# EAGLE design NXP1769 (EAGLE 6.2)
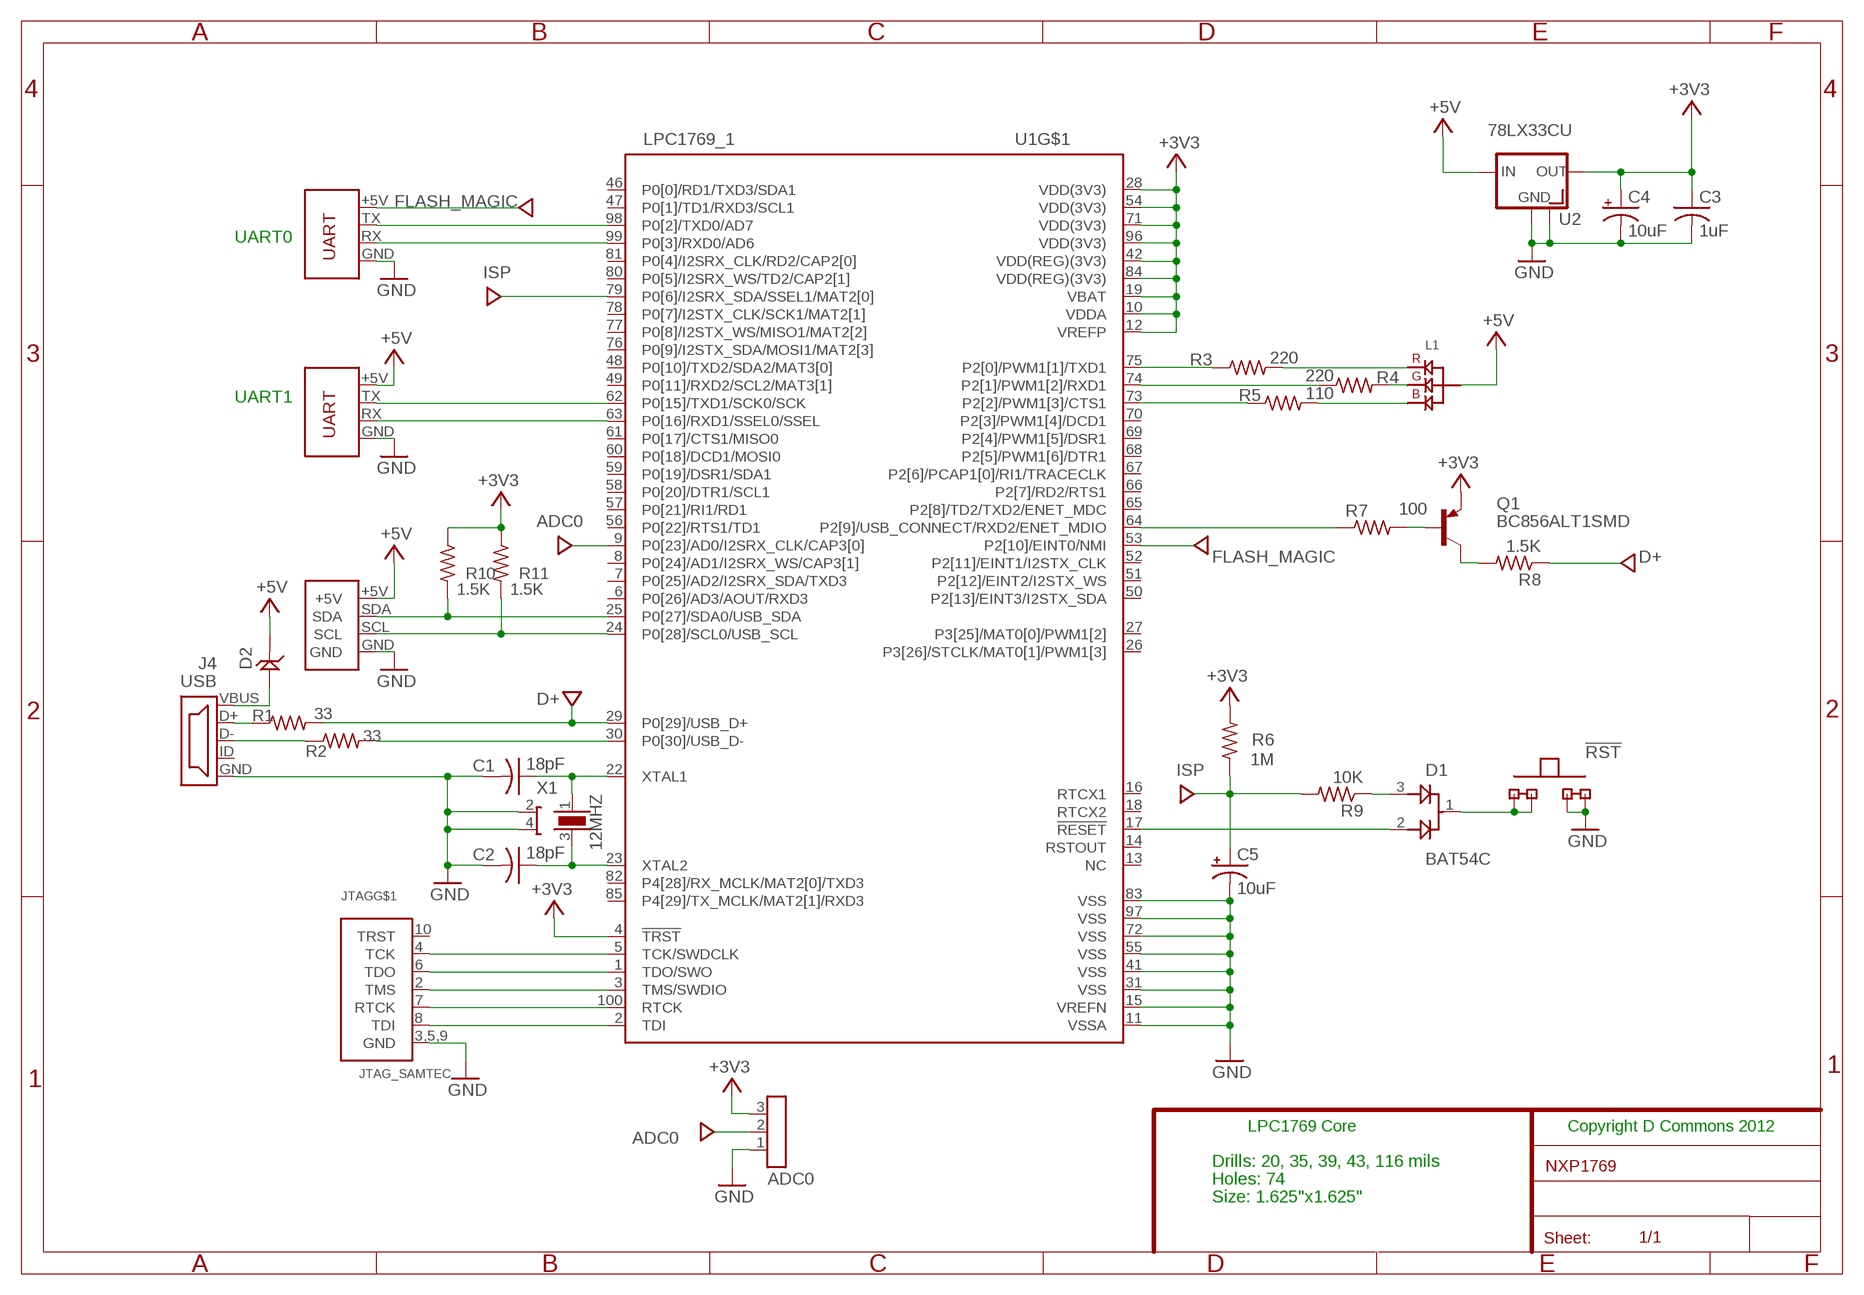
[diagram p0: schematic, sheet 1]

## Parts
!RST  SIDE_SWITCH  [COLLISION]
ADC0  1X3  [1X03]
C1  18pF  C-USC0805  [C0805]
C2  18pF  C-USC0805  [C0805]
C3  1uF  C-USC0805  [C0805]
C4  10uF  C_POL1206  [C1206P]
C5  10uF  C_POL1206  [C1206P]
D1  BAT54C  [SOT23-BAT54C]
D2  PMEG2005  [SOT23]
J1  ISNAP  [ISNAP]
J4  USB  [USB-MB-S]
JTAG  JTAG_SAMTEC  [2X10X0.5MM]
L1  RGB_ANODE  [3.2X2.7]
Q1  BC856ALT1SMD  [SOT23-BEC]
R1  33  R-US_R0805  [R0805]
R2  33  R-US_R0805  [R0805]
R3  220  R-US_R0805  [R0805]
R4  220  R-US_R0805  [R0805]
R5  110  R-US_R0805  [R0805]
R6  1M  R-US_R0805  [R0805]
R7  100  R-US_R0805  [R0805]
R8  1.5K  R-US_R0805  [R0805]
R9  10K  R-US_R0805  [R0805]
R10  1.5K  R-US_R0805  [R0805]
R11  1.5K  R-US_R0805  [R0805]
U1  LPC1769_1  [LQFP100-14X14]
U2  78LX33CU  [SOT89]
UART0  IMU_UART  [IMU_UART]
UART1  IMU_UART  [IMU_UART]
X1  12MHZ  16MHZ  [3.2X2.5_XTAL]

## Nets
!RESET: D1.2 U1.17(!RESET)
!RST_SW: !RST.A !RST.A@1(A) D1.1
+3V3 [+3V3]: ADC0.3 C3.1 C4.+ Q1.E R6.2 R10.1 R11.1 U1.4(!TRST) U1.10(VDDA) U1.12(VREFP) U1.19(VBAT) U1.28(VDD(3V3)) U1.42(VDD(REG)(3V3)) U1.54(VDD(3V3)) U1.71(VDD(3V3)) U1.84(VDD(REG)(3V3)) U1.96(VDD(3V3)) U2.1(OUT)
+5V [+5V]: D2.3(CATHODE) J1.+5V L1.A U2.3(IN) UART1.+5V
ADC0: ADC0.2 U1.9(P0[23]/AD0/I2SRX_CLK/CAP3[0])
BLUE: L1.B R5.2
D+: R1.2 R8.1 U1.29(P0[29]/USB_D+)
D-: R2.2 U1.30(P0[30]/USB_D-)
DD+: J4.D+ R1.1
DD-: J4.D- R2.1
FLASH_MAGIC: U1.53(P2[10]/EINT0/NMI) UART0.+5V
GND: !RST.B !RST.B@1(B) ADC0.1 C1.2 C2.2 C3.2 C4.- C5.- J1.GND J4.GND JTAG.3,5,9(GND) U1.11(VSSA) U1.15(VREFN) U1.31(VSS) U1.41(VSS) U1.55(VSS) U1.72(VSS) U1.83(VSS) U1.97(VSS) U2.2(GND) U2.4(GND1) UART0.GND UART1.GND X1.2(GND) X1.4(GND)
GREEN: L1.G R4.2
ISP: C5.+ R6.1 R9.2 U1.79(P0[6]/I2SRX_SDA/SSEL1/MAT2[0])
N$24: Q1.B R7.2
N$25: Q1.C R8.2
N$28: D1.3 R9.1
P2.0: R3.1 U1.75(P2[0]/PWM1[1]/TXD1)
P2.1: R4.1 U1.74(P2[1]/PWM1[2]/RXD1)
P2.2: R5.1 U1.73(P2[2]/PWM1[3]/CTS1)
RED: L1.R R3.2
RTCK: JTAG.7(RTCK) U1.100(RTCK)
RXD0: U1.99(P0[3]/RXD0/AD6) UART0.RX
RXD1: U1.63(P0[16]/RXD1/SSEL0/SSEL) UART1.RX
SCL: J1.SCL R11.2 U1.24(P0[28]/SCL0/USB_SCL)
SDA: J1.SDA R10.2 U1.25(P0[27]/SDA0/USB_SDA)
TCK: JTAG.4(TCK) U1.5(TCK/SWDCLK)
TDI: JTAG.8(TDI) U1.2(TDI)
TDO: JTAG.6(TDO) U1.1(TDO/SWO)
TMS: JTAG.2(TMS) U1.3(TMS/SWDIO)
TXD0: U1.98(P0[2]/TXD0/AD7) UART0.TX
TXD1: U1.62(P0[15]/TXD1/SCK0/SCK) UART1.TX
USB_EN: R7.1 U1.64(P2[9]/USB_CONNECT/RXD2/ENET_MDIO)
VBUS: D2.1(ANODE) J4.VBUS
XTAL1: C1.1 U1.22(XTAL1) X1.1(X0)
XTAL2: C2.1 U1.23(XTAL2) X1.3(X1)
Unconnected: J4.ID(UID) JTAG.10(TRST) U1.6(P0[26]/AD3/AOUT/RXD3) U1.7(P0[25]/AD2/I2SRX_SDA/TXD3) U1.8(P0[24]/AD1/I2SRX_WS/CAP3[1]) U1.13(NC) U1.14(RSTOUT) U1.16(RTCX1) U1.18(RTCX2) U1.20(P1[31]/SCK1/AD05) U1.21(P1[30]/AD4) U1.26(P3[26]/STCLK/MAT0[1]/PWM1[3]) U1.27(P3[25]/MAT0[0]/PWM1[2]) U1.32(P1[18]/PWM1[1]/CAP1[0]) U1.33(P1[19]/MCOA0/USB_PPWR/CAP1[1]) U1.34(P1[20]/MCI0/PWM1[2]/SCK0) U1.35(P1[21]/MCABORT/PWM1[3]/SSEL0) U1.36(P1[22]/MCOB0/MAT1[0]) U1.37(P1[23]/MCI1/PWM1[4]/MISO0) U1.38(P1[24]/MCI2/PWM1[5]/MOSI0) U1.39(P1[25]/MCOA1/MAT1[1]) U1.40(P1[26]/MCOB1/PWM1[6]/CAP0[0]) U1.43(P1[27]/CLKOUT/CAP0[1]) U1.44(P1[28]/MCOA2/PCAP1[0]/MAT0[0]) U1.45(P1[29]/MCOB2/PCAP1[1]/MAT0[1]) U1.46(P0[0]/RD1/TXD3/SDA1) U1.47(P0[1]/TD1/RXD3/SCL1) U1.48(P0[10]/TXD2/SDA2/MAT3[0]) U1.49(P0[11]/RXD2/SCL2/MAT3[1]) U1.50(P2[13]/EINT3/I2STX_SDA) U1.51(P2[12]/EINT2/I2STX_WS) U1.52(P2[11]/EINT1/I2STX_CLK) U1.56(P0[22]/RTS1/TD1) U1.57(P0[21]/RI1/RD1) U1.58(P0[20]/DTR1/SCL1) U1.59(P0[19]/DSR1/SDA1) U1.60(P0[18]/DCD1/MOSI0) U1.61(P0[17]/CTS1/MISO0) U1.65(P2[8]/TD2/TXD2/ENET_MDC) U1.66(P2[7]/RD2/RTS1) U1.67(P2[6]/PCAP1[0]/RI1/TRACECLK) U1.68(P2[5]/PWM1[6]/DTR1) U1.69(P2[4]/PWM1[5]/DSR1) U1.70(P2[3]/PWM1[4]/DCD1) U1.76(P0[9]/I2STX_SDA/MOSI1/MAT2[3]) U1.77(P0[8]/I2STX_WS/MISO1/MAT2[2]) U1.78(P0[7]/I2STX_CLK/SCK1/MAT2[1]) U1.80(P0[5]/I2SRX_WS/TD2/CAP2[1]) U1.81(P0[4]/I2SRX_CLK/RD2/CAP2[0]) U1.82(P4[28]/RX_MCLK/MAT2[0]/TXD3) U1.85(P4[29]/TX_MCLK/MAT2[1]/RXD3) U1.86(P1[17]/ENET_MDIO) U1.87(P1[16]/ENET_MDC) U1.88(P1[15]/ENET_REF_CLK) U1.89(P1[14]/ENET_RX_ER) U1.90(P1[10]/ENET_RXD1) U1.91(P1[9]/ENET_RXD0) U1.92(P1[8]/ENET_CRS) U1.93(P1[4]/ENET_TX_EN) U1.94(P1[1]/ENET_TXD1) U1.95(P1[0]/ENET_TXD0)

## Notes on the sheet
- UART0
- UART1
- LPC1769 Core | Copyright D Commons 2012
- Drills: 20, 35, 39, 43, 116 mils
- Holes: 74
- Size: 1.625"x1.625"

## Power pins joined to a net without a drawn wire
GND: J4.GND@1(GND) J4.GND@2(GND) J4.GND@3(GND) J4.GND@4(GND) JTAG.3,5,9@1(GND) JTAG.3,5,9@2(GND)

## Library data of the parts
!RST = 1_Motor:SIDE_SWITCH
ADC0 = 1_Dougs_custom:1X3
C1-C3 = 1_Dougs_custom:C-US: CAPACITOR, American symbol
C4 C5 = 1_Dougs_custom:C_POL1206
D1 = 1_Dougs_custom:BAT54C
D2 = 1_Dougs_custom:PMEG2005
J1 = 1_Dougs_custom:ISNAP
J4 = 1_Dougs_custom:USB: USB Connectors
JTAG = 1_Dougs_custom:JTAG_SAMTEC
L1 = 1_Dougs_custom:RGB_ANODE
Q1 = transistor-pnp:BC856*: PNP Transistror
R1-R11 = 1_Dougs_custom:R-US_: RESISTOR, American symbol
U1 = 1_linux:LPC1769_1: LPC1768 100 MHz 32-bit ARM Cortex-M3 based microcontroller featuring a high level of integration and low power consumption. 512 kB Flash, 64 kB SRAM, USB Device/Host/OTG, 2 CAN, DAC, Ethernet MarcVl - Datasheet available on www.nxp.com
U2 = 1_Dougs_custom:78LX33CU: VOLTAGE REGULATOR
UART0 UART1 = 1_Dougs_custom:IMU_UART
X1 = RF_lib:16MHZ

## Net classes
1 +5V: width 0.381 mm
2 +3V3: width 0.229 mm

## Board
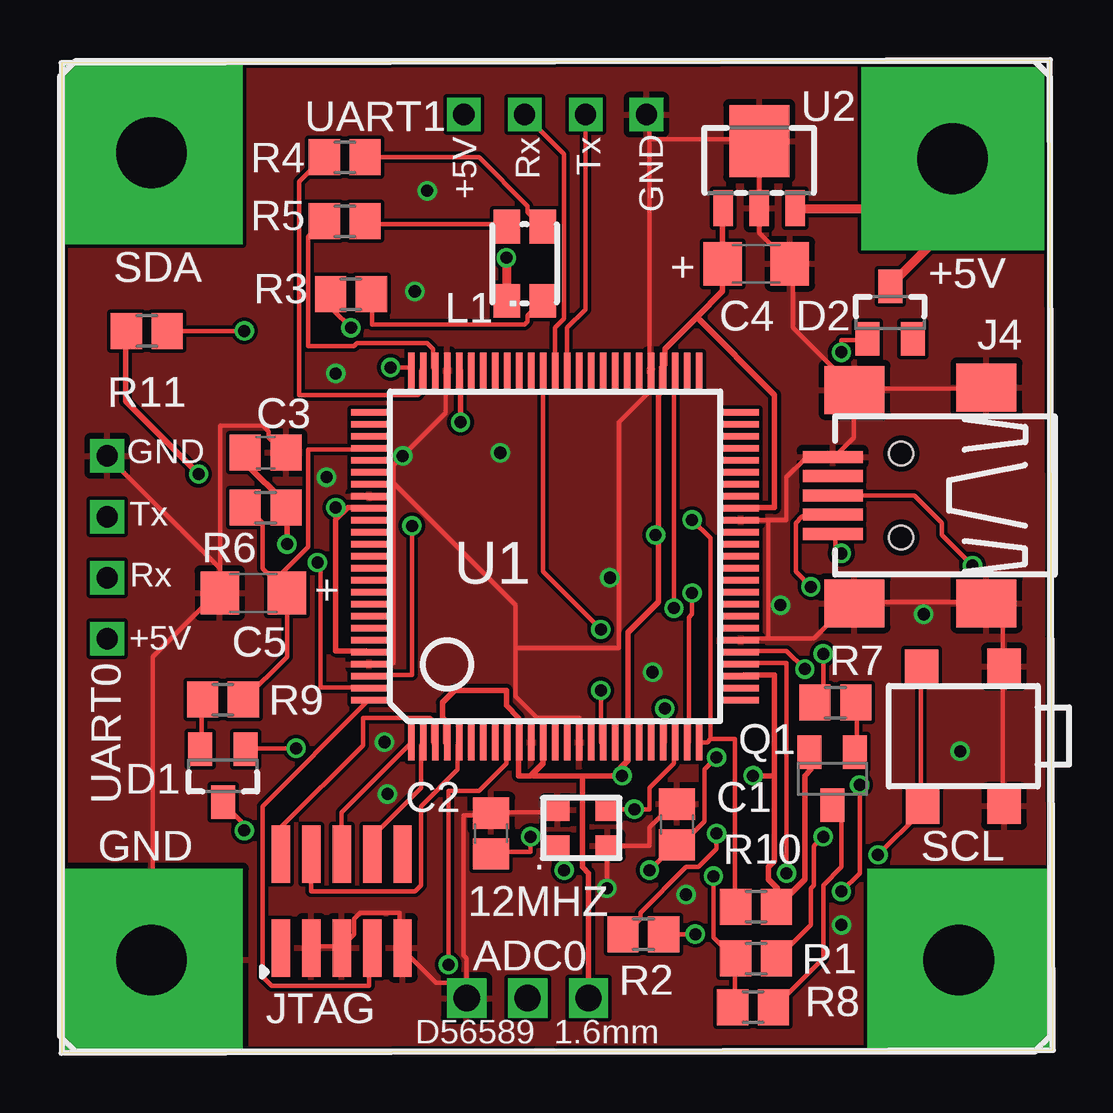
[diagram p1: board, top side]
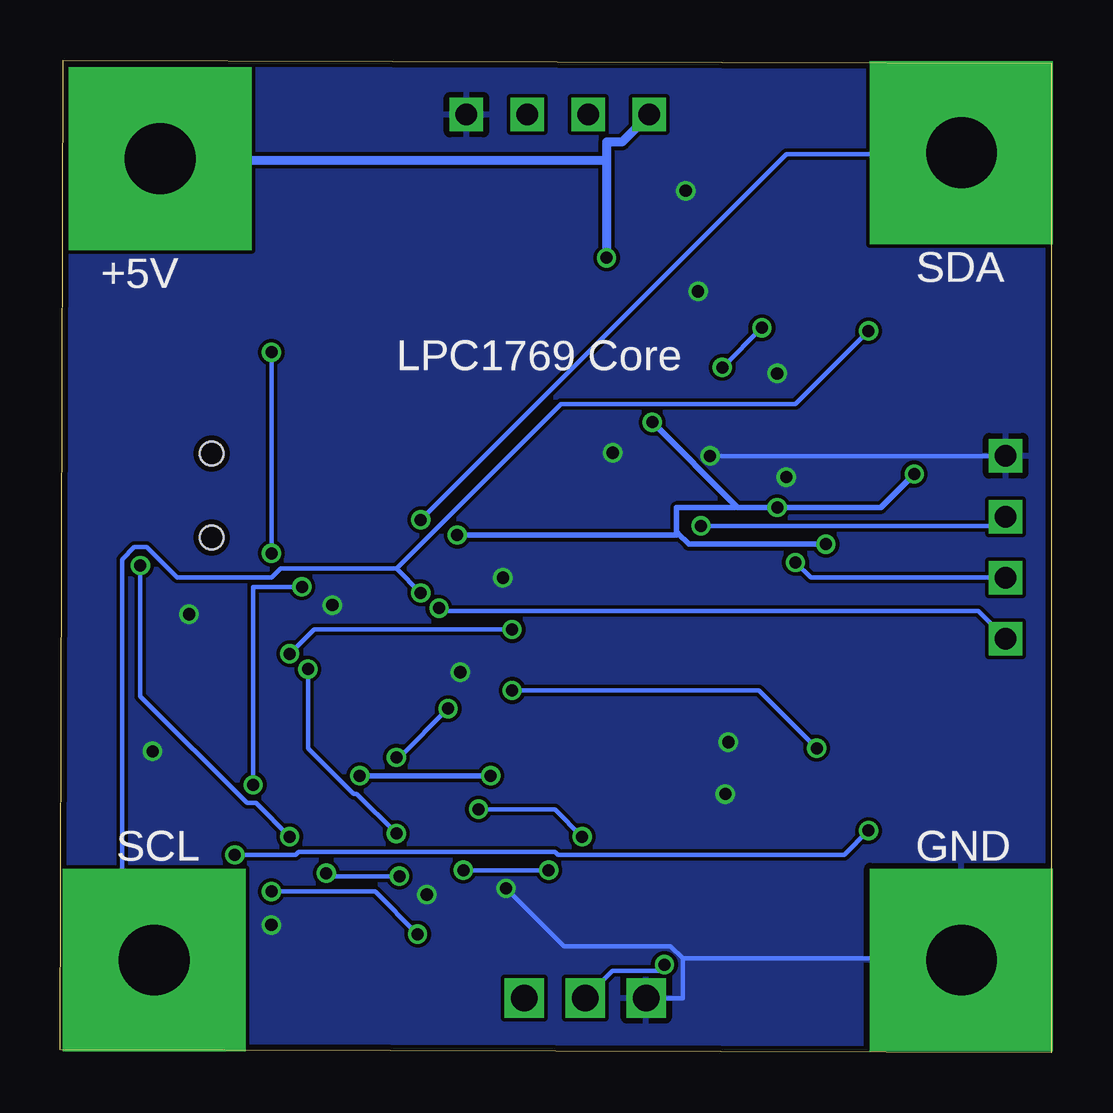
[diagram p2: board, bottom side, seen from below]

Size 41.33 x 41.39 mm. Coordinates in mm from the lower left corner, seen from the top.
Outline: 0,0 41.33,0.13 41.2,41.39 0,41.27 0,0
Copper layers (1*16): Top 0.035mm / dielectric 1.5mm / Bottom 0.035mm
Design rules: minimum track width 6mil, minimum drill 12mil, track to track 6mil, track to pad 6mil, pad to pad 6mil, via to via 6mil, smd to smd 0mil, copper to edge 10mil, drill to drill 10mil, minimum pad ring 10mil, minimum via ring 6mil, stop-mask expansion 2mil, vias tented up to drill 100mil, thermal gap 10mil

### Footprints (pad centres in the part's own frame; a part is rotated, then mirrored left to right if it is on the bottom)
COLLISION = smd 1.5 x 1.4: A 2.87,1.74; A@1 -2.9,1.7; B 2.9,-1.7; B@1 -2.91,-1.7
1X03 = drill 1.092 square: 1 -2.54,0; 2 0,0; 3 2.54,0
C0805 = smd 1.3 x 1.5: 1 -0.85,0; 2 0.85,0
C1206P = smd 1.6 x 1.8: + 1.4,0; - -1.4,0
SOT23-BAT54C = smd 1 x 1.4: 1 0,1.1; 2 -0.95,-1.1; 3 0.95,-1.1
SOT23 = smd 1 x 1.4: 1 -0.95,-1.1; 2 0.95,-1.1; 3 0,1.1
ISNAP = drill 2.946 pad 7.62 square: +5V 16.573,16.573; GND -16.828,-16.828; SCL 16.828,-16.828; SDA -16.828,16.828
USB-MB-S = smd 0.5 x 2.5: D+ 0,-9.25; D- 0.8,-9.25; GND -1.6,-9.25; ID -0.8,-9.25; VBUS 1.6,-9.25 | smd 2 x 2.5: GND@1 4.5,-2.842; GND@2 4.5,-8.342; GND@3 -4.5,-2.842; GND@4 -4.4,-8.342 | hole 0.991: -1.75,-6.4; 1.75,-6.4
2X10X0.5MM = smd 0.76 x 2.4: 2 0.38,5.11; 3,5,9 1.65,1.2; 3,5,9@1 2.92,1.2; 3,5,9@2 5.46,1.2; 4 1.65,5.11; 6 2.92,5.11; 7 4.19,1.2; 8 4.19,5.11; 10 5.46,5.11; NC 0.38,1.2
3.2X2.7 = smd 1.4 x 1.1: A 1.55,-0.75; B -1.55,-0.75; G -1.55,0.75; R 1.55,0.75
SOT23-BEC = smd 1 x 1.4: B -0.95,-1.1; C 0,1.1; E 0.95,-1.1
R0805 = smd 1.3 x 1.5: 1 -0.85,0; 2 0.85,0
LQFP100-14X14 = smd 0.27 x 1.5: 1 -6,-7.75; 2 -5.5,-7.75; 3 -5,-7.75; 4 -4.5,-7.75; 5 -4,-7.75; 6 -3.5,-7.75; 7 -3,-7.75; 8 -2.5,-7.75; 9 -2,-7.75; 10 -1.5,-7.75; 11 -1,-7.75; 12 -0.5,-7.75; 13 0,-7.75; 14 0.5,-7.75; 15 1,-7.75; 16 1.5,-7.75; 17 2,-7.75; 18 2.5,-7.75; 19 3,-7.75; 20 3.5,-7.75; 21 4,-7.75; 22 4.5,-7.75; 23 5,-7.75; 24 5.5,-7.75; 25 6,-7.75; 51 6,7.75; 52 5.5,7.75; 53 5,7.75; 54 4.5,7.75; 55 4,7.75; 56 3.5,7.75; 57 3,7.75; 58 2.5,7.75; 59 2,7.75; 60 1.5,7.75; 61 1,7.75; 62 0.5,7.75; 63 0,7.75; 64 -0.5,7.75; 65 -1,7.75; 66 -1.5,7.75; 67 -2,7.75; 68 -2.5,7.75; 69 -3,7.75; 70 -3.5,7.75; 71 -4,7.75; 72 -4.5,7.75; 73 -5,7.75; 74 -5.5,7.75; 75 -6,7.75 | smd 1.5 x 0.27: 26 7.75,-6; 27 7.75,-5.5; 28 7.75,-5; 29 7.75,-4.5; 30 7.75,-4; 31 7.75,-3.5; 32 7.75,-3; 33 7.75,-2.5; 34 7.75,-2; 35 7.75,-1.5; 36 7.75,-1; 37 7.75,-0.5; 38 7.75,0; 39 7.75,0.5; 40 7.75,1; 41 7.75,1.5; 42 7.75,2; 43 7.75,2.5; 44 7.75,3; 45 7.75,3.5; 46 7.75,4; 47 7.75,4.5; 48 7.75,5; 49 7.75,5.5; 50 7.75,6; 76 -7.75,6; 77 -7.75,5.5; 78 -7.75,5; 79 -7.75,4.5; 80 -7.75,4; 81 -7.75,3.5; 82 -7.75,3; 83 -7.75,2.5; 84 -7.75,2; 85 -7.75,1.5; 86 -7.75,1; 87 -7.75,0.5; 88 -7.75,0; 89 -7.75,-0.5; 90 -7.75,-1; 91 -7.75,-1.5; 92 -7.75,-2; 93 -7.75,-2.5; 94 -7.75,-3; 95 -7.75,-3.5; 96 -7.75,-4; 97 -7.75,-4.5; 98 -7.75,-5; 99 -7.75,-5.5; 100 -7.75,-6
SOT89 = smd 0.8 x 1.5: 1 -1.5,-1.75; 2 0,-1.75; 3 1.5,-1.75 | smd 2.5 x 3: 4 0,1.05
IMU_UART = drill 0.889 square: +5V 0,3.81; GND 0,-3.81; RX 0,1.27; TX 0,-1.27
3.2X2.5_XTAL = smd 1 x 0.9: 1 0.6,0.5; 2 2.7,0.5; 3 2.7,2; 4 0.6,2

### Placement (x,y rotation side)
!RST  37.59,13.21 90 top
ADC0  19.43,2.29 0 top
C1  25.65,9.53 90 top
C2  17.91,9.14 90 top
C3  8.51,25.02 0 top
C4  28.96,32.89 180 top
C5  8,19.18 0 top
D1  6.73,11.56 180 top
D2  34.54,30.86 0 top
J1  20.57,20.7 0 top
J4  41.4,23.24 270 top
JTAG  8.76,3.17 0 top
L1  19.3,32.89 270 top
Q1  32.13,11.43 180 top
R1  28.96,3.94 180 top
R2  24.26,4.95 180 top
R3  12.06,31.62 0 top
R4  11.81,37.34 0 top
R5  11.81,34.67 0 top
R6  8.51,22.73 0 top
R7  32.26,14.61 0 top
R8  28.83,1.91 0 top
R9  6.73,14.73 0 top
R10  28.96,6.1 180 top
R11  3.56,30.1 0 top
U1  20.57,20.7 0 top
U2  29.08,36.96 0 top
UART0  1.91,21.08 180 top
UART1  20.57,39.12 90 top
X1  20.07,8.13 0 top

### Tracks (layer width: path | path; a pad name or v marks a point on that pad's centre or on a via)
!RESET  (via drill 0.5)
  Top 0.178: v9.78,12.7 7.75,12.7 D1.2 | v22.48,15.11 22.48,12.95 U1.17
  Bottom 0.178: v9.78,12.7 12.19,15.11 v22.48,15.11
!RST_SW  (via drill 0.5)
  Top 0.178: v7.62,9.27 7.62,9.53 6.73,10.41 D1.1 | v34.04,8.26 35.81,10.03 35.81,10.29 !RST.A@1 35.81,10.41 35.81,16 !RST.A
  Bottom 0.178: v7.62,9.27 8.64,8.26 20.57,8.26 20.7,8.38 31.37,8.38 31.5,8.26 v34.04,8.26
+3V3  (via drill 0.5)
  Top 0.229: 9.4,22.73 9.4,22.86 7.62,24.64 7.62,25.02 C3.1 | 11.49,22.29 11.94,22.73 12.7,22.73 U1.84 | 11.49,22.29 11.43,22.22 11.43,16.76 12.7,16.76 U1.96 | v16.64,26.29 16.64,28.45 U1.71 | v11.43,22.73 11.43,22.35 11.49,22.29 | v5.71,24.13 2.67,27.18 2.67,30.1 R11.1 | v9.4,21.21 9.4,22.73 | 9.4,22.73 R6.2 | 26.48,30.67 27.56,31.75 C4.+ | 26.48,30.67 25.15,29.34 25.15,28.7 25.02,28.57 U1.54 25.02,28.45 25.02,27.56 24.89,27.43 24.89,21.59 | 26.48,30.67 29.72,27.43 29.72,22.73 28.45,22.73 U1.42 | C4.+ 27.56,35.18 U2.1 | C4.+ | 29.84,6.22 29.97,6.22 30.99,7.24 30.99,11.56 31.24,11.81 31.24,12.45 Q1.E | 29.84,6.22 29.84,6.1 R10.1 29.84,6.22 | 29.72,11.56 29.72,8 29.46,7.75 29.46,7.24 29.84,6.86 29.84,6.22 | 29.72,11.56 29.72,15.75 28.45,15.75 U1.28 | U1.4 16,12.95 16,13.84 15.88,13.97 15.88,14.61 16.38,15.11 18.54,15.11 18.54,14.48 19.05,13.97 19.05,12.95 U1.10 19.05,12.83 19.05,11.56 19.56,11.56 19.62,11.62 | 19.62,11.62 20.07,12.07 20.07,12.83 U1.12 | 23.18,11.75 22.99,11.56 21.72,11.56 | 23.18,11.75 23.62,12.19 23.62,12.83 U1.19 23.62,12.95 23.62,17.53 24.89,18.8 24.89,21.59 | 21.72,11.56 19.68,11.56 19.62,11.62 | ADC0.3 21.97,7.49 21.72,7.75 21.72,11.56 | v28.83,11.56 29.72,11.56 | 23.18,11.75 v23.37,11.56 | 24.89,21.59 v24.77,21.59
  Bottom 0.229: 13.14,22.8 13.08,22.73 v11.43,22.73 7.11,22.73 v5.71,24.13 | 13.14,22.8 v16.64,26.29 | v9.4,21.21 15.11,21.21 15.56,21.65 | 15.56,21.65 15.62,21.72 15.62,22.73 13.21,22.73 13.14,22.8 | v23.37,11.56 v28.83,11.56 | v24.77,21.59 15.62,21.59 15.56,21.65
+5V  (via drill 0.5)
  Top 0.381: v18.54,33.15 18.54,31.37 L1.A | D2.3 34.54,32 37.08,34.54 37.08,37.21 J1.+5V 36.96,35.18 30.61,35.18 U2.3
  Bottom 0.381: 18.54,37.21 18.54,37.97 17.91,37.97 UART1.+5V | 18.54,37.21 v18.54,33.15 | 18.54,37.21 37.08,37.21 J1.+5V
ADC0  (via drill 0.5)
  Top 0.178: v16.13,3.68 16.13,10.92 17.4,10.92 18.54,12.07 18.54,12.83 U1.9
  Bottom 0.178: v16.13,3.68 16.38,3.43 18.29,3.43 ADC0.2
BLUE
  Top 0.178: L1.B 18.54,34.54 12.7,34.54 12.7,34.67 R5.2
D+  (via drill 0.5)
  Top 0.178: 28.07,3.94 28.07,1.91 R8.1 | v30.23,7.49 30.23,16.26 28.45,16.26 U1.29 | v27.18,7.37 27.18,4.83 28.07,3.94 | 28.07,3.94 R1.2
  Bottom 0.178: v30.23,7.49 30.1,7.37 v27.18,7.37
D-  (via drill 0.5)
  Top 0.178: v27.3,9.14 27.3,8.51 26.54,7.75 26.04,7.75 24.13,5.84 24.13,5.59 23.5,4.95 R2.2 | v30.99,16 30.23,16.76 28.45,16.76 U1.30
  Bottom 0.178: v27.3,9.14 28.96,10.79 29.08,10.79 30.99,12.7 v30.99,16
DD+  (via drill 0.5)
  Top 0.178: v31.75,9.02 31.37,8.64 31.37,6.98 31.24,6.86 31.24,5.33 29.84,3.94 R1.1 | v37.97,20.32 36.7,21.59 36.7,22.1 35.56,23.24 J4.D+
  Bottom 0.178: v31.75,9.02 33.15,10.41 33.53,10.41 37.97,14.86 v37.97,20.32
DD-  (via drill 0.5)
  Top 0.178: v26.42,4.95 R2.1 | v32.51,6.73 33.27,7.49 v33.27,11.18 | v31.24,19.43 30.61,20.07 30.61,22.1 30.86,22.35 32.13,22.35 J4.D-
  Bottom 0.178: v26.42,4.95 28.19,6.73 v32.51,6.73 | v33.27,11.18 33.27,19.43 v31.24,19.43
FLASH_MAGIC  (via drill 0.5)
  Top 0.178: v25.53,18.54 25.53,28.45 U1.53
  Bottom 0.178: v25.53,18.54 25.4,18.41 3.05,18.41 UART0.+5V
GND  (via drill 0.5, 0.51)
  Top 0.178: 19.81,13.97 19.56,13.72 19.56,12.95 U1.11 | 19.81,13.97 21.59,13.97 21.59,12.95 U1.15 | 13.84,22.99 13.84,16.26 12.83,16.26 U1.97 | 13.84,22.99 13.72,23.11 12.83,23.11 U1.83 | 13.84,22.99 13.84,23.75 | 13.84,23.75 13.84,24.51 v14.22,24.89 16,26.67 16,28.45 U1.72 | 19.81,13.97 18.92,14.86 18.92,16.89 | 18.92,16.89 18.92,18.67 13.84,23.75 | 29.46,17.27 31.37,17.27 32.77,18.67 33.02,18.67 J4.GND@2 33.15,18.8 38.48,18.8 J4.GND@1 38.61,18.67 39.24,18.03 39.24,16.13 !RST.B 39.24,16 39.24,10.41 !RST.B@1 | 29.46,17.27 28.45,17.27 U1.31 | 29.46,22.22 28.45,22.22 U1.41 | 29.46,17.27 29.46,22.22 | J4.GND@4 33.02,27.56 33.02,25.65 32.26,24.89 J4.GND 32.13,24.77 30.99,24.77 30.23,24 30.23,22.22 29.46,22.22 | J4.GND@3 38.48,27.69 33.15,27.69 J4.GND@4 | 24.51,38.1 24.51,38.99 UART1.GND | 24.51,38.1 24.51,28.57 U1.55 24.51,28.45 24.51,27.56 23.24,26.29 23.24,16.89 18.92,16.89 | 24.51,38.1 29.08,38.1 U2.4 U2.2 29.08,34.16 C4.- 30.48,32.89 30.48,30.23 33.02,27.69 J4.GND@4 | JTAG.3,5,9 10.41,4.44 11.56,4.44 JTAG.3,5,9@1 11.68,4.44 12.19,4.95 12.19,5.59 12.45,5.84 14.1,5.84 14.1,4.44 JTAG.3,5,9@2 14.22,4.32 15.62,2.92 16.89,2.92 | C1.2 25.65,10.29 25.4,10.29 24.51,9.4 24.51,8.64 22.86,8.64 X1.2 22.73,8.51 v22.73,6.86 | X1.4 20.57,10.03 17.91,10.03 C2.2 17.91,9.91 16.76,9.91 16.76,4.06 16.89,3.94 16.89,2.92 | 16.89,2.92 ADC0.1 | 6.6,20.19 C5.- 6.48,19.18 3.81,16.51 3.81,3.94 J1.GND | 6.6,20.19 6.6,26.16 8.38,26.16 8.64,25.91 8.64,25.65 9.27,25.02 C3.2 | 6.6,20.19 UART0.GND
  Bottom 0.178: v22.73,6.86 20.32,4.44 15.88,4.44 15.37,3.94 | 15.37,3.94 15.37,2.29 ADC0.1 | 15.37,3.94 3.81,3.94 J1.GND | UART0.GND v14.22,24.89
  other vias: 14.73,31.75 15.24,35.94 18.29,25.02 35.94,18.29 22.86,19.81 11.43,28.32 11.05,24 13.46,12.95 24.64,15.88 32.51,5.33 13.59,10.79 26.04,6.6 29.97,18.67 37.47,12.57
  pour Bottom: 0,0.13 41.15,0.13 41.15,41.4 0,41.4
  pour Top: 0,0.13 41.27,0.13 41.27,41.4 0,41.4
GREEN
  Top 0.178: R4.2 17.4,37.34 19.43,35.31 19.43,35.05 19.94,34.54 L1.G
ISP
  Top 0.178: C5.+ 9.4,16.51 7.62,14.73 R9.2 | C5.+ 8.89,19.68 | 8.89,19.68 8.38,20.19 8.38,22.1 7.75,22.73 R6.1 | C5.+ 8.89,19.68 | 8.89,19.68 10.29,21.08 10.29,25.15 12.7,25.15 U1.79
N$24
  Top 0.178: Q1.B 33.15,12.57 33.15,14.61 R7.2
N$25
  Top 0.178: Q1.C 32.13,10.29 32.51,9.91 32.51,7.75 31.75,6.98 31.75,3.94 29.72,1.91 R8.2
N$28
  Top 0.178: D1.3 5.84,12.7 5.84,14.73 R9.1
P2.0  (via drill 0.5)
  Top 0.178: v13.72,28.57 14.48,28.57 U1.75 | v12.06,30.23 11.3,30.99 11.3,31.62 R3.1
  Bottom 0.178: v12.06,30.23 v13.72,28.57
P2.1
  Top 0.178: U1.74 14.99,28.45 14.99,27.56 14.86,27.43 9.91,27.43 9.91,36.32 10.92,37.34 R4.1
P2.2
  Top 0.178: U1.73 15.49,28.57 15.49,29.34 15.24,29.59 12.32,29.59 12.19,29.46 10.29,29.46 10.29,34.04 10.92,34.67 R5.1
RED
  Top 0.178: L1.R 19.94,31.24 19.43,30.73 19.43,30.48 19.3,30.35 12.95,30.35 12.95,31.62 R3.2
RTCK
  Top 0.178: U1.100 12.7,14.61 8.38,10.29 8.38,3.17 8.76,2.79 12.83,2.79 12.83,4.32 JTAG.7
RXD0  (via drill 0.5)
  Top 0.178: v10.67,20.45 10.79,20.32 10.79,15.24 12.7,15.24 U1.99
  Bottom 0.178: v10.67,20.45 10.03,19.81 UART0.RX
RXD1
  Top 0.178: U1.63 20.57,30.23 20.95,30.61 20.95,37.47 UART1.RX
SCL  (via drill 0.5)
  Top 0.178: v26.29,19.18 26.29,18.29 26.16,18.16 26.16,12.95 U1.24 | v7.62,30.1 R11.2
  Bottom 0.178: 27.3,20.19 v26.29,19.18 | 27.3,20.19 32.13,20.19 32.51,19.81 36.45,19.81 37.72,21.08 38.23,21.08 38.73,20.57 38.73,3.94 37.47,3.94 J1.SCL | v7.62,30.1 10.67,27.05 20.45,27.05 27.3,20.19
SDA  (via drill 0.5)
  Top 0.178: 27.05,13.08 26.92,12.95 26.67,12.95 U1.25 | 27.05,13.08 28.07,13.08 28.07,6.1 R10.2 | 27.05,13.08 27.05,21.46 v26.29,22.22
  Bottom 0.178: v26.29,22.22 11.05,37.47 3.81,37.47 J1.SDA
TCK
  Top 0.178: U1.5 16.51,12.83 16.51,11.81 14.99,10.29 14.99,6.98 14.73,6.73 10.41,6.73 10.41,8.26 JTAG.4
TDI
  Top 0.178: U1.2 14.99,12.83 14.99,11.05 12.95,9.02 12.95,8.38 JTAG.8
TDO
  Top 0.178: U1.1 14.48,12.83 11.68,10.03 11.68,8.38 JTAG.6
TMS
  Top 0.178: U1.3 15.49,12.95 15.49,13.84 15.37,13.97 12.57,13.97 12.57,12.83 9.14,9.4 9.14,8.38 JTAG.2
TXD0  (via drill 0.5)
  Top 0.178: v14.61,21.97 14.61,15.75 12.83,15.75 U1.98
  Bottom 0.178: v14.61,21.97 2.29,21.97 UART0.TX
TXD1
  Top 0.178: UART1.TX 21.84,30.99 21.08,30.23 21.08,28.57 U1.62
USB_EN  (via drill 0.5)
  Top 0.178: v31.75,16.64 31.75,14.86 31.5,14.61 R7.1 | v22.48,17.65 20.07,20.07 U1.64
  Bottom 0.178: v31.75,16.64 30.73,17.65 v22.48,17.65
VBUS  (via drill 0.5)
  Top 0.178: v32.51,29.21 32.51,29.72 33.53,29.72 D2.1 | v32.51,20.83 32.26,21.08 32.26,21.59 J4.VBUS
  Bottom 0.178: v32.51,20.83 v32.51,29.21
XTAL1  (via drill 0.5)
  Top 0.178: v20.95,7.62 20.95,8.26 20.7,8.51 X1.1 | 25.65,8.76 v24.51,7.62 | v25.15,14.35 25.15,12.95 U1.22 | v27.3,12.32 26.8,11.81 26.8,9.65 25.91,8.76 25.65,8.76 | 25.65,8.76 C1.1
  Bottom 0.178: v24.51,7.62 v20.95,7.62 | v25.15,14.35 27.18,12.32 v27.3,12.32
XTAL2  (via drill 0.5)
  Top 0.178: X1.3 22.86,10.16 v23.88,10.16 24.51,10.16 24.51,11.05 25.53,12.07 25.53,12.83 U1.23 | v19.56,9.02 19.56,8.38 17.91,8.38 C2.1
  Bottom 0.178: v19.56,9.02 20.7,10.16 v23.88,10.16

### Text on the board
tPlace: D56589_1.6mm
bPlace: LPC1769 Core
_tplace: U2 | UART1 | +5V | GND | R4 | Rx | Tx | R5 | + | SDA | +5V | R3 | . | C4 | L1 | D2 | J4 | R11 | C3 | GND | Tx | U1 | Rx | R6 | + | +5V | C5 | R7 | R9 | Q1 | D1 | C2 | UART0 | C1 | R10 | GND | . | SCL | 12MHZ | R2 | R1 | ADC0 | JTAG | R8
_bplace: SDA | +5V | LPC1769 Core | GND | SCL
